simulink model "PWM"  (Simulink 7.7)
settings: Solver=ode5  StartTime=0.0  StopTime=0.002  FixedStep=0.00001  RelTol=1e-3
InitFcn:
  | GNM_lsg_ini
StopFcn:
  | PWM_plot
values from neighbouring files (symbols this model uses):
  Fpwm = 5000    [GNM_lsg_ini.m]
  Umax = 200    [GNM_lsg_ini.m]
libraries: simulink x1

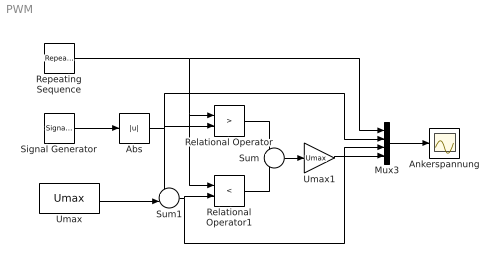
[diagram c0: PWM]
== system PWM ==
  Abs : Abs
  Ankerspannung : Scope
  Mux3 : Mux
  Relational Operator : RelationalOperator  Operator=>
  Relational Operator1 : RelationalOperator  Operator=<
  Repeating Sequence : simulink/Sources/Repeating Sequence  SystemSampleTime=-1  rep_seq_t=[0 2.1] * 0.001  rep_seq_y=[0.9 -0.4] * Umax
  Signal Generator : SignalGenerator  WaveForm=sawtooth  Amplitude=Umax  Frequency=Fpwm
  Sum : Sum  Inputs=+-
  Sum1 : Sum  Inputs=+-|
  Umax : Constant  Value=Umax
  Umax1 : Gain  Gain=Umax
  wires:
  Repeating Sequence/1 -> Relational Operator/1, Relational Operator1/1, Mux3/1
  Abs/1 -> Sum1/1, Relational Operator/2, Mux3/2
  Umax/1 -> Sum1/2
  Relational Operator/1 -> Sum/1
  Relational Operator1/1 -> Sum/2
  Sum/1 -> Umax1/1
  Mux3/1 -> Ankerspannung/1
  Umax1/1 -> Mux3/4
  Sum1/1 -> Relational Operator1/2, Mux3/3
  Signal Generator/1 -> Abs/1
